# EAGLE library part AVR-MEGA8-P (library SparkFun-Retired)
MCU 8 Kbytes FLASH 1 kbytes SRAM 512 bytes EEPROM USART 6-channel 10 bit ADC 2-channel 8 bit ADC SparkFun Products None.
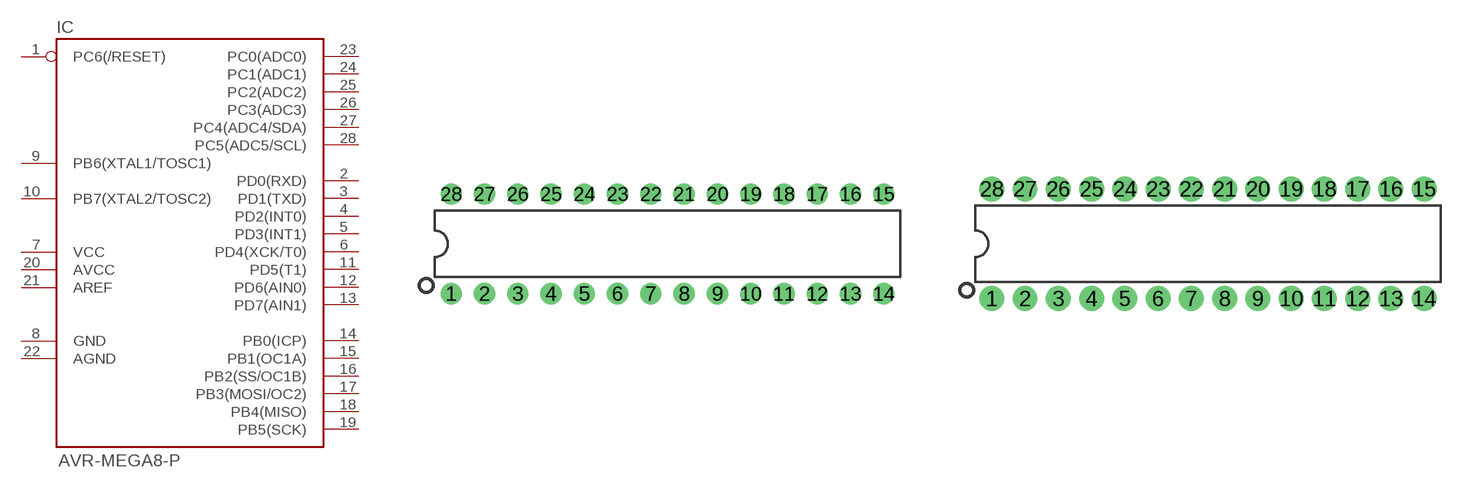
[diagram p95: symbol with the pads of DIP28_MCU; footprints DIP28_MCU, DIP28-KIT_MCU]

Designator prefix IC

## AVR-MEGA8-PPTH  [DIP28_MCU]
1  PC6(/RESET)
2  PD0(RXD)
3  PD1(TXD)
4  PD2(INT0)
5  PD3(INT1)
6  PD4(XCK/T0)
7  VCC
8  GND
9  PB6(XTAL1/TOSC1)
10  PB7(XTAL2/TOSC2)
11  PD5(T1)
12  PD6(AIN0)
13  PD7(AIN1)
14  PB0(ICP)
15  PB1(OC1A)
16  PB2(SS/OC1B)
17  PB3(MOSI/OC2)
18  PB4(MISO)
19  PB5(SCK)
20  AVCC
21  AREF
22  AGND
23  PC0(ADC0)
24  PC1(ADC1)
25  PC2(ADC2)
26  PC3(ADC3)
27  PC4(ADC4/SDA)
28  PC5(ADC5/SCL)

## AVR-MEGA8-PSIM  [DIP28-KIT_MCU]
Pads as for DIP28_MCU

## AVR-MEGA8-PZIF_SOCKET  [DIL28-ZIF_SOCKET_MCU]
Pads as for DIP28_MCU

## Footprint DIP28_MCU (pad centres in mm)
Standard 28-pin DIP package. IC needs to have legs bent before insertion.
drill 0.813 pad 1.626: 1 -16.51,-3.81; 2 -13.97,-3.81; 3 -11.43,-3.81; 4 -8.89,-3.81; 5 -6.35,-3.81; 6 -3.81,-3.81; 7 -1.27,-3.81; 8 1.27,-3.81; 9 3.81,-3.81; 10 6.35,-3.81; 11 8.89,-3.81; 12 11.43,-3.81; 13 13.97,-3.81; 14 16.51,-3.81; 15 16.51,3.81; 16 13.97,3.81; 17 11.43,3.81; 18 8.89,3.81; 19 6.35,3.81; 20 3.81,3.81; 21 1.27,3.81; 22 -1.27,3.81; 23 -3.81,3.81; 24 -6.35,3.81; 25 -8.89,3.81; 26 -11.43,3.81; 27 -13.97,3.81; 28 -16.51,3.81

## Footprint DIP28-KIT_MCU (pad centres in mm)
drill 0.864 pad 1.905: 1 -16.51,-4.191; 2 -13.97,-4.191; 3 -11.43,-4.191; 4 -8.89,-4.191; 5 -6.35,-4.191; 6 -3.81,-4.191; 7 -1.27,-4.191; 8 1.27,-4.191; 9 3.81,-4.191; 10 6.35,-4.191; 11 8.89,-4.191; 12 11.43,-4.191; 13 13.97,-4.191; 14 16.51,-4.191; 15 16.51,4.191; 16 13.97,4.191; 17 11.43,4.191; 18 8.89,4.191; 19 6.35,4.191; 20 3.81,4.191; 21 1.27,4.191; 22 -1.27,4.191; 23 -3.81,4.191; 24 -6.35,4.191; 25 -8.89,4.191; 26 -11.43,4.191; 27 -13.97,4.191; 28 -16.51,4.191

## Footprint DIL28-ZIF_SOCKET_MCU (pad centres in mm)
drill 1.016 pad 1.88: 1 -16.51,-3.81; 2 -13.97,-3.81; 3 -11.43,-3.81; 4 -8.89,-3.81; 5 -6.35,-3.81; 6 -3.81,-3.81; 7 -1.27,-3.81; 8 1.27,-3.81; 9 3.81,-3.81; 10 6.35,-3.81; 11 8.89,-3.81; 12 11.43,-3.81; 13 13.97,-3.81; 14 16.51,-3.81; 15 16.51,3.81; 16 13.97,3.81; 17 11.43,3.81; 18 8.89,3.81; 19 6.35,3.81; 20 3.81,3.81; 21 1.27,3.81; 22 -1.27,3.81; 23 -3.81,3.81; 24 -6.35,3.81; 25 -8.89,3.81; 26 -11.43,3.81; 27 -13.97,3.81; 28 -16.51,3.81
